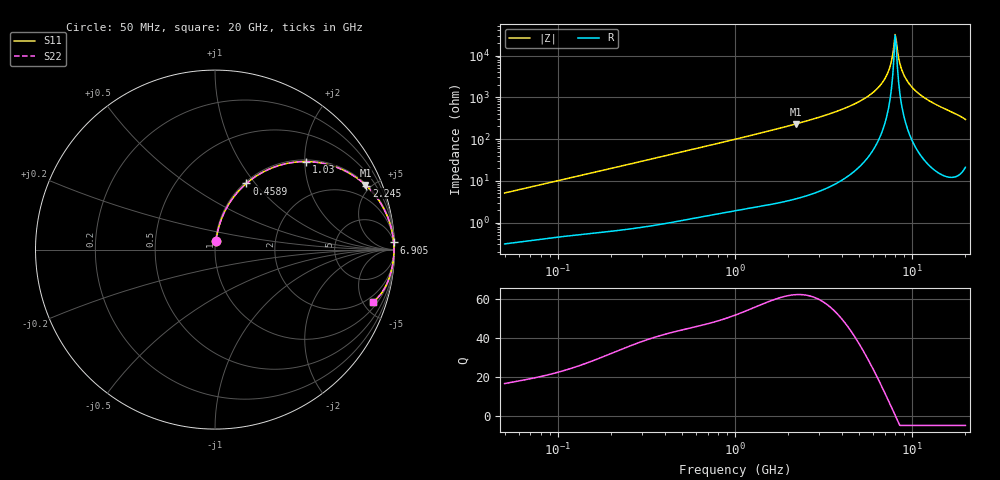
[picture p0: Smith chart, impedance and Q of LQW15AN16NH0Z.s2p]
!Murata Part Number: LQW15AN16NH0Z
!These Parameters are Measured in Series Mode Connection
!  o--[Z]--o
!Port1  Port2
!  o-------o
!Freq. Start=50[MHz] Stop=20[GHz], 401[Steps]
# Hz S RI R 50
!Freq.(Hz) S11(Real) S11(Imag) S21(Real) S21(Imag) S12(Real) S12(Imag) S22(Real) S22(Imag)
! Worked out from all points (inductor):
!   401 points, 50 MHz to 20 GHz, reference 50 ohm
!   read as one part in series: L = 16.1 nH near 51.52 MHz
!   highest Q = 62.3 at 2.212 GHz (marker M1), where L = 16.6 nH
!   self-resonance near 8.021 GHz
!   S11 on the Smith chart (normalised r, x): 50 MHz: 1.01, +0.10; 458.9 MHz: 1.02, +0.90; 1.03 GHz: 1.04, +2.03; 2.245 GHz: 1.08, +4.70; 6.905 GHz: 5, +50; 20 GHz: 1.42, -5.89
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5e7  0.00563 0.0505  0.9944 -0.0505  0.9944 -0.0505  0.00563 0.0505
1.364002e8  0.023 0.132  0.977 -0.132  0.977 -0.132  0.023 0.132
3.721004e8  0.1243 0.318  0.8757 -0.318  0.8757 -0.318  0.1243 0.318
4.589149e8  0.1749 0.3685  0.8251 -0.3685  0.8251 -0.3685  0.1749 0.3685
1e9  0.4933 0.4904  0.5067 -0.4904  0.5067 -0.4904  0.4933 0.4904
1.030411e9  0.5083 0.4904  0.4917 -0.4904  0.4917 -0.4904  0.5083 0.4904
2.211938e9  0.8379 0.3606  0.1621 -0.3606  0.1621 -0.3606  0.8379 0.3606
2.245319e9  0.8425 0.3563  0.1575 -0.3563  0.1575 -0.3563  0.8425 0.3563
2.728004e9  0.8942 0.2995  0.1058 -0.2995  0.1058 -0.2995  0.8942 0.2995
5.041459e9  0.9812 0.1228  0.0188 -0.1228  0.0188 -0.1228  0.9812 0.1228
6.034176e9  0.9912 0.0749  0.00882 -0.0749  0.00882 -0.0749  0.9912 0.0749
6.905011e9  0.9954 0.0397  0.00463 -0.0397  0.00463 -0.0397  0.9954 0.0397
7.442007e9  0.9966 0.0203  0.00343 -0.0203  0.00343 -0.0203  0.9966 0.0203
7.901521e9  0.997 0.00475  0.00302 -0.00475  0.00302 -0.00475  0.997 0.00475
8.141811e9  0.997 -0.00301  0.003 0.00301  0.003 0.00301  0.997 -0.00301
8.264682e9  0.997 -0.0069  0.00304 0.0069  0.00304 0.0069  0.997 -0.0069
8.644534e9  0.9967 -0.0186  0.00334 0.0186  0.00334 0.0186  0.9967 -0.0186
8.907419e9  0.9963 -0.0264  0.00369 0.0264  0.00369 0.0264  0.9963 -0.0264
9.457416e9  0.9952 -0.0422  0.0048 0.0422  0.0048 0.0422  0.9952 -0.0422
1.019291e10  0.9931 -0.0621  0.00694 0.0621  0.00694 0.0621  0.9931 -0.0621
1.276073e10  0.9807 -0.1247  0.0193 0.1247  0.0193 0.1247  0.9807 -0.1247
2e10  0.8805 -0.2905  0.1195 0.2905  0.1195 0.2905  0.8805 -0.2905
